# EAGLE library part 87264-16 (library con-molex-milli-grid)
RECEPTACAL
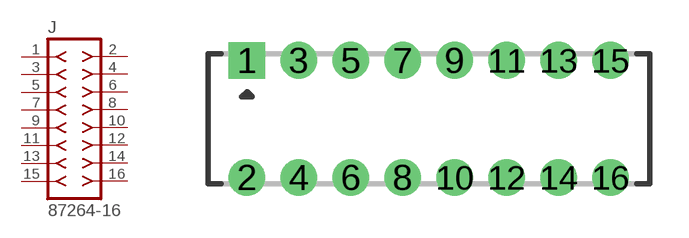
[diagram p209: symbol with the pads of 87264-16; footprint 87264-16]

Designator prefix J

## 87264-16  [87264-16]
1  1  pas
2  2  pas
3  3  pas
4  4  pas
5  5  pas
6  6  pas
7  7  pas
8  8  pas
9  9  pas
10  10  pas
11  11  pas
12  12  pas
13  13  pas
14  14  pas
15  15  pas
16  16  pas

## Footprint 87264-16 (pad centres in mm)
RECEPTACAL Dual Row, Side Entry
drill 0.914 square: 1 -7,2.25
drill 0.914: 2 -7,-2.25; 3 -5,2.25; 4 -5,-2.25; 5 -3,2.25; 6 -3,-2.25; 7 -1,2.25; 8 -1,-2.25; 9 1,2.25; 10 1,-2.25; 11 3,2.25; 12 3,-2.25; 13 5,2.25; 14 5,-2.25; 15 7,2.25; 16 7,-2.25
